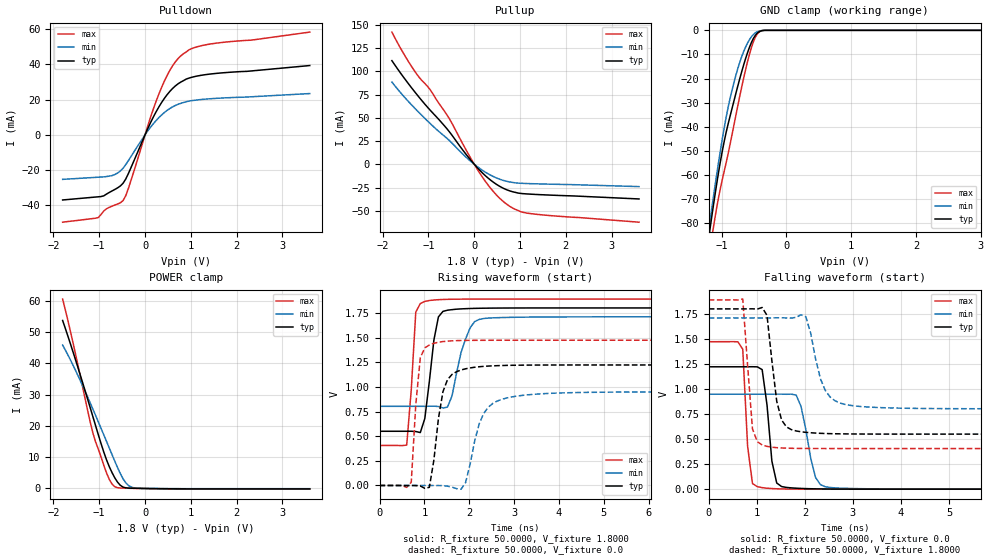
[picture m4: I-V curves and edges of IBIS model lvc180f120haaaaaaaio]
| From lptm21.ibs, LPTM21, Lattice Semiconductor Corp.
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|   Model lvc180f120haaaaaaaio
[Model]   lvc180f120haaaaaaaio
Model_type   I/O
Polarity   Non-Inverting
Enable   Active-Low
Vinl =   0.6300V
Vinh =   1.1700V
Vmeas =   0.9000V
Cref =   0.0F
Rref =   1.0000M
Vref =   0.0V
C_comp   4.2000pF   3.8000pF   7.5000pF
[Temperature Range]   25.0000   0.1050k   -40.0000
[Voltage Range]   1.8000V   1.7100V   1.8900V
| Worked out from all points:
|   slope of the pulldown table from 0 to 0.27 V, typ, clamps not added: 18.8 ohm
|   slope of the pullup table from 0 to 0.27 V, typ, clamps not added: 20.1 ohm
|   GND clamp passes 1 mA (typ) near -0.44 V on its own axis
|   POWER clamp passes 1 mA (typ) near -0.54 V on its own axis
|   rising waveform, R_fixture 50.0000, V_fixture 1.8000: 20-80 % time 202ps typ, 308ps min, 128ps max; typ from 0.55 V to 1.8 V
|   rising waveform, R_fixture 50.0000, V_fixture 0.0: 20-80 % time 229ps typ, 363ps min, 143ps max; typ from 0 V to 1.22 V
|   falling waveform, R_fixture 50.0000, V_fixture 0.0: 20-80 % time 157ps typ, 235ps min, 114ps max; typ from 1.22 V to 0 V
|   falling waveform, R_fixture 50.0000, V_fixture 1.8000: 20-80 % time 203ps typ, 295ps min, 139ps max; typ from 1.8 V to 0.55 V
[Pulldown]
|Voltage   I(typ)   I(min)   I(max)
-1.8V     -36.96mA   -25.25mA   -49.57mA
-1.02V    -35.15mA   -24.02mA   -46.92mA
-900mV    -34.59mA   -23.83mA   -43.17mA
-720mV    -31.83mA   -23.11mA   -40.45mA
-480mV    -27.47mA   -18.92mA   -37.31mA
-360mV    -21.77mA   -14.48mA   -30.15mA
120mV     6.916mA    4.342mA    9.968mA
360mV     18.31mA    11.28mA    26.84mA
600mV     26.32mA    15.89mA    39.15mA
840mV     30.81mA    18.38mA    46.1mA
1.38V     34.43mA    20.45mA    51.43mA
3.6V      39.4mA     23.48mA    58.4mA
[Pullup]
|Voltage   I(typ)   I(min)   I(max)
-1.8V     111.4mA    88.42mA    142.1mA
-1.56V    94.6mA     74.12mA    120.4mA
-1.32V    79.08mA    61.28mA    101.4mA
-960mV    57.98mA    43.63mA    79.88mA
-600mV    38.35mA    28.07mA    53.32mA
-120mV    7.04mA     4.994mA    10.22mA
120mV     -6.437mA   -4.482mA   -9.543mA
300mV     -14.76mA   -10.17mA   -22.19mA
660mV     -26.37mA   -17.71mA   -41.08mA
900mV     -30.25mA   -20.01mA   -48.54mA
1.2V      -32.04mA   -20.78mA   -52.84mA
3.6V      -37.29mA   -24.01mA   -62.27mA
[GND_clamp]
|Voltage   I(typ)   I(min)   I(max)
-1.8V     -240.1mA   -229.3mA   -254.1mA
-1.2V     -86.06mA   -82.86mA   -94.69mA
-1.17V    -80.34mA   -77.04mA   -89.11mA
-1.11V    -69.35mA   -65.72mA   -78.69mA
-1.02V    -54.38mA   -49.81mA   -65.51mA
-930mV    -42.15mA   -35.85mA   -54.74mA
-780mV    -26.05mA   -18.53mA   -35.08mA
-690mV    -17.04mA   -10.83mA   -23.36mA
-570mV    -6.946mA   -3.801mA   -9.827mA
-450mV    -1.119mA   -561.2uA   -1.47mA
-330mV    0A         -3.874uA   0A
3.6V      0A         0A         0A
[POWER_clamp]
|Voltage   I(typ)   I(min)   I(max)
-1.8V     53.66mA    45.8mA     60.51mA
-1.62V    45.76mA    40.78mA    49.57mA
-1.26V    28.84mA    29.42mA    25.34mA
-1.14V    22.99mA    25.38mA    17.77mA
-960mV    14.31mA    19.19mA    10.02mA
-840mV    9.109mA    15mA       4.931mA
-720mV    5.041mA    10.79mA    1.399mA
-660mV    3.38mA     8.712mA    551.7uA
-540mV    1.01mA     4.773mA    153.1uA
-420mV    197.6uA    1.797mA    88.49uA
-240mV    59.36uA    194.4uA    21.2uA
3.6V      -132uA     -74.33uA   -225.9uA
[Ramp]
| variable   typ   min   max
dV/dt_r  0.7331/0.2268n   0.5691/0.3594n   0.8835/0.1420n
dV/dt_f  0.7502/0.2007n   0.5444/0.2916n   0.8906/0.1381n
R_load = 50.0000
[Rising Waveform]
R_fixture=   50.0000
V_fixture=   1.8000
V_fixture_min=   1.7100
V_fixture_max=   1.8900
|time   V(typ)   V(min)   V(max)
0s        549.6mV    802.6mV    405.7mV
606.1ps   549.6mV    802.6mV    409.8mV
808.1ps   547.2mV    802.6mV    1.758V
1.01ns    679.3mV    802.6mV    1.866V
1.212ns   1.474V     804.2mV    1.88V
1.414ns   1.765V     785.4mV    1.886V
1.616ns   1.783V     908.3mV    1.888V
2.02ns    1.794V     1.599V     1.89V
2.222ns   1.797V     1.684V     1.89V
10ns      1.8V       1.71V      1.89V
[Rising Waveform]
R_fixture=   50.0000
V_fixture=   0.0
V_fixture_min=   0.0
V_fixture_max=   0.0
|time   V(typ)   V(min)   V(max)
0s        335.1nV    508.3nV    248.8nV
707.1ps   -57.36uV   614.4nV    32.97mV
909.1ps   -4.993mV   13.4uV     1.296V
1.111ns   -18.57mV   11.2uV     1.424V
1.212ns   258.9mV    -255.2uV   1.442V
1.414ns   951.4mV    -1.605mV   1.459V
1.919ns   1.183V     30mV       1.471V
2.323ns   1.208V     731mV      1.472V
2.828ns   1.218V     886.2mV    1.472V
10ns      1.222V     948.4mV    1.472V
[Falling Waveform]
R_fixture=   50.0000
V_fixture=   0.0
V_fixture_min=   0.0
V_fixture_max=   0.0
|time   V(typ)   V(min)   V(max)
0s        1.222V     948.4mV    1.472V
707.1ps   1.222V     948.4mV    1.397V
808.1ps   1.222V     948.4mV    427.5mV
1.01ns    1.221V     948.4mV    24.99mV
1.111ns   1.193V     948.4mV    15.28mV
1.313ns   279.8mV    948.5mV    6.02mV
1.515ns   26.18mV    948.9mV    2.383mV
1.818ns   9.629mV    939mV      586.8uV
2.424ns   1.858mV    24.36mV    67.33uV
10ns      -7.862uV   -27.3uV    22uV
[Falling Waveform]
R_fixture=   50.0000
V_fixture=   1.8000
V_fixture_min=   1.7100
V_fixture_max=   1.8900
|time   V(typ)   V(min)   V(max)
0s        1.8V       1.71V      1.89V
707.1ps   1.8V       1.71V      1.898V
909.1ps   1.801V     1.71V      601.8mV
1.111ns   1.814V     1.71V      441.1mV
1.414ns   877.3mV    1.711V     414.3mV
1.717ns   594.6mV    1.708V     408.1mV
2.02ns    567.4mV    1.721V     406.3mV
2.424ns   555.7mV    985.7mV    405.8mV
2.828ns   551.9mV    847mV      405.7mV
10ns      549.6mV    802.7mV    405.7mV
